(* Logix 5000 Module export GRACO_PD2K; software revision 32.04 *)

MODULES
   GRACO_PD2K : ETHERNET-MODULE (Ethernet 192.168.1.50, rev 1.1, Output RPI 100 ms)   // Graco Example PD2K
        GRACO_PD2K:I   // PD2K1 module status
        GRACO_PD2K:I.DATA[0]   // PD2K1 mix unit 1 system mode
        GRACO_PD2K:I.DATA[1]   // PD2K1 mix unit 1 event flag
        GRACO_PD2K:I.DATA[2]   // PD2K1 mix unit 1 actual mix flow/pressure (cc/min in flow mode, psi in pressure mode)
        GRACO_PD2K:I.DATA[3]   // PD2K1 mix unit 1 actual mix ratio (A*100 : B)
        GRACO_PD2K:I.DATA[4]   // PD2K1 mix unit 1 actual pot life remaining (sec)
        GRACO_PD2K:I.DATA[5]   // PD2K1 mix unit 1 gun 1 trigger status
        GRACO_PD2K:I.DATA[6]   // PD2K1 mix unit 1 pump 1 status
        GRACO_PD2K:I.DATA[7]   // PD2K1 mix unit 1 pump 2 status
        GRACO_PD2K:I.DATA[8]   // PD2K1 mix unit 1 pump 1 current material
        GRACO_PD2K:I.DATA[9]   // PD2K1 mix unit 1 pump 2 current material
        GRACO_PD2K:I.DATA[10]   // PD2K1 mix unit 1 actual pump 1 flow rate (cc/min)
        GRACO_PD2K:I.DATA[11]   // PD2K1 mix unit 1 actual pump 2 flow rate (cc/min)
        GRACO_PD2K:I.DATA[12]   // PD2K1 mix unit 1 actual pump 1 pressure (psi)
        GRACO_PD2K:I.DATA[13]   // PD2K1 mix unit 1 actual pump 2 pressure (psi)
        GRACO_PD2K:I.DATA[14]   // PD2K1 mix unit 1 active recipe number
        GRACO_PD2K:I.DATA[15]   // PD2K1 mix unit 1 active recipe material A
        GRACO_PD2K:I.DATA[16]   // PD2K1 mix unit 1 active recipe material B
        GRACO_PD2K:I.DATA[17]   // PD2K1 mix unit 1 active recipe flush sequence A
        GRACO_PD2K:I.DATA[18]   // PD2K1 mix unit 1 active recipe flush sequence B
        GRACO_PD2K:I.DATA[19]   // PD2K1 mix unit 1 active mix ratio SP (A*100 : B)
        GRACO_PD2K:I.DATA[20]   // PD2K1 mix unit 1 active pot life time SP (min)
        GRACO_PD2K:I.DATA[21]   // PD2K1 mix unit 1 active job number
        GRACO_PD2K:I.DATA[22]   // PD2K1 mix unit 1 job material A sprayed volume (cc)
        GRACO_PD2K:I.DATA[23]   // PD2K1 mix unit 1 job material B sprayed volume (cc)
        GRACO_PD2K:I.DATA[24]   // PD2K1 mix unit 1 job material solvent sprayed volume (cc)
        GRACO_PD2K:I.DATA[25]   // PD2K1 mix unit 1 safety interlock status
        GRACO_PD2K:I.DATA[26]   // PD2K1 mix unit 2 system mode
        GRACO_PD2K:I.DATA[27]   // PD2K1 mix unit 2 event flag
        GRACO_PD2K:I.DATA[28]   // PD2K1 mix unit 2 actual mix flow/pressure (cc/min in flow mode, psi in pressure mode)
        GRACO_PD2K:I.DATA[29]   // PD2K1 mix unit 2 actual mix ratio (A*100 : B)
        GRACO_PD2K:I.DATA[30]   // PD2K1 mix unit 2 actual pot life remaining (sec)
        GRACO_PD2K:I.DATA[31]   // PD2K1 mix unit 2 gun 2 trigger status
        GRACO_PD2K:I.DATA[32]   // PD2K1 mix unit 2 pump 3 status
        GRACO_PD2K:I.DATA[33]   // PD2K1 mix unit 2 pump 4 status
        GRACO_PD2K:I.DATA[34]   // PD2K1 mix unit 2 pump 3 current material
        GRACO_PD2K:I.DATA[35]   // PD2K1 mix unit 2 pump 4 current material
        GRACO_PD2K:I.DATA[36]   // PD2K1 mix unit 2 actual pump 3 flow rate (cc/min)
        GRACO_PD2K:I.DATA[37]   // PD2K1 mix unit 2 actual pump 4 flow rate (cc/min)
        GRACO_PD2K:I.DATA[38]   // PD2K1 mix unit 2 actual pump 3 pressure (psi)
        GRACO_PD2K:I.DATA[39]   // PD2K1 mix unit 2 actual pump 4 pressure (psi)
        GRACO_PD2K:I.DATA[40]   // PD2K1 mix unit 2 active recipe number
        GRACO_PD2K:I.DATA[41]   // PD2K1 mix unit 2 active recipe material A
        GRACO_PD2K:I.DATA[42]   // PD2K1 mix unit 2 active recipe material B
        GRACO_PD2K:I.DATA[43]   // PD2K1 mix unit 2 active recipe flush sequence A
        GRACO_PD2K:I.DATA[44]   // PD2K1 mix unit 2 active recipe flush sequence B
        GRACO_PD2K:I.DATA[45]   // PD2K1 mix unit 2 active mix ratio SP (A*100 : B)
        GRACO_PD2K:I.DATA[46]   // PD2K1 mix unit 2 active pot life time SP (min)
        GRACO_PD2K:I.DATA[47]   // PD2K1 mix unit 2 active job number
        GRACO_PD2K:I.DATA[48]   // PD2K1 mix unit 2 job material A sprayed volume (cc)
        GRACO_PD2K:I.DATA[49]   // PD2K1 mix unit 2 job material B sprayed volume (cc)
        GRACO_PD2K:I.DATA[50]   // PD2K1 mix unit 2 job material solvent sprayed volume (cc)
        GRACO_PD2K:I.DATA[51]   // PD2K1 mix unit 2 safety interlock status
        GRACO_PD2K:I.DATA[52]   // PD2K1 DCS return 0
        GRACO_PD2K:I.DATA[53]   // PD2K1 DCS return 1
        GRACO_PD2K:I.DATA[54]   // PD2K1 DCS return 2
        GRACO_PD2K:I.DATA[55]   // PD2K1 DCS return 3
        GRACO_PD2K:I.DATA[56]   // PD2K1 DCS return 4
        GRACO_PD2K:I.DATA[57]   // PD2K1 DCS return 5
        GRACO_PD2K:I.DATA[58]   // PD2K1 DCS return 6
        GRACO_PD2K:I.DATA[59]   // PD2K1 DCS return 7
        GRACO_PD2K:I.DATA[60]   // PD2K1 DCS return 8
        GRACO_PD2K:I.DATA[61]   // PD2K1 DCS acknowledge
        GRACO_PD2K:O   // PD2K1 module commands
        GRACO_PD2K:O.DATA[0]   // PD2K1 mix unit 1 system mode command
        GRACO_PD2K:O.DATA[1]   // PD2K1 mix unit 1 clear active alarm/deviation
        GRACO_PD2K:O.DATA[2]   // PD2K1 mix unit 1 goto recipe number
        GRACO_PD2K:O.DATA[3]   // PD2K1 mix unit 1 mix control setpoint (cc/min in flow mode, psi in pressure mode)
        GRACO_PD2K:O.DATA[4]   // PD2K1 mix unit 1 mix fill setpoint (cc/min in flow mode, psi in pressure mode)
        GRACO_PD2K:O.DATA[5]   // PD2K1 mix unit 1 pump flush sequence number / prime material number
        GRACO_PD2K:O.DATA[6]   // PD2K1 mix unit 1 pump flush/prime command
        GRACO_PD2K:O.DATA[7]   // PD2K1 mix unit 1 job complete command
        GRACO_PD2K:O.DATA[8]   // PD2K1 mix unit 1 gun 1 trigger
        GRACO_PD2K:O.DATA[9]   // PD2K1 mix unit 1 fluid control mode (0=flow, 1=pressure)
        GRACO_PD2K:O.DATA[10]   // PD2K1 mix unit 2 system mode command
        GRACO_PD2K:O.DATA[11]   // PD2K1 mix unit 2 clear active alarm/deviation
        GRACO_PD2K:O.DATA[12]   // PD2K1 mix unit 2 goto recipe number
        GRACO_PD2K:O.DATA[13]   // PD2K1 mix unit 2 mix control setpoint (cc/min in flow mode, psi in pressure mode)
        GRACO_PD2K:O.DATA[14]   // PD2K1 mix unit 2 mix fill setpoint (cc/min in flow mode, psi in pressure mode)
        GRACO_PD2K:O.DATA[15]   // PD2K1 mix unit 2 pump flush sequence number / prime material number
        GRACO_PD2K:O.DATA[16]   // PD2K1 mix unit 2 pump flush/prime command
        GRACO_PD2K:O.DATA[17]   // PD2K1 mix unit 2 job complete command
        GRACO_PD2K:O.DATA[18]   // PD2K1 mix unit 2 gun 2 trigger
        GRACO_PD2K:O.DATA[19]   // PD2K1 mix unit 2 fluid control mode (0=flow, 1=pressure)
        GRACO_PD2K:O.DATA[20]   // PD2K1 DCS argument 0
        GRACO_PD2K:O.DATA[21]   // PD2K1 DCS argument 1
        GRACO_PD2K:O.DATA[22]   // PD2K1 DCS argument 2
        GRACO_PD2K:O.DATA[23]   // PD2K1 DCS argument 3
        GRACO_PD2K:O.DATA[24]   // PD2K1 DCS argument 4
        GRACO_PD2K:O.DATA[25]   // PD2K1 DCS argument 5
        GRACO_PD2K:O.DATA[26]   // PD2K1 DCS argument 6
        GRACO_PD2K:O.DATA[27]   // PD2K1 DCS argument 7
        GRACO_PD2K:O.DATA[28]   // PD2K1 DCS argument 8
        GRACO_PD2K:O.DATA[29]   // PD2K1 DCS command
        GRACO_PD2K:C   // PD2K1 module configuration
END_MODULES
